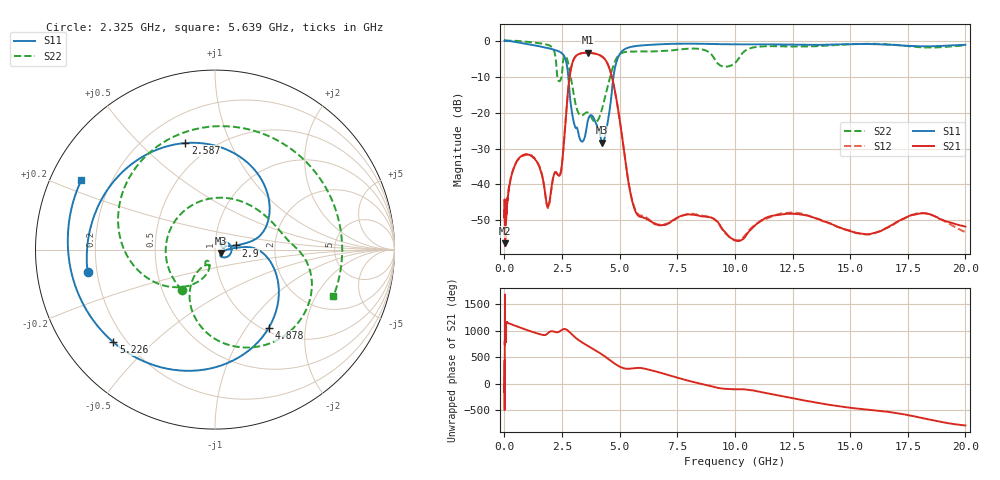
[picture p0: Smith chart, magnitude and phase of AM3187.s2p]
!Agilent Technologies,E8364B,MY43040894,A.07.50.67
!Agilent E8364B: A.07.50.67
!Date: Friday, December 27, 2019 08:39:41
!Correction: S11(Full 2 Port(1,2))
!S21(Full 2 Port(1,2))
!S12(Full 2 Port(1,2))
!S22(Full 2 Port(1,2))
!S2P File: Measurements: S11, S21, S12, S22:Log Frequency Sweep
# Hz S  dB  R 50
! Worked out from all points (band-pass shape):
!   3201 points, 10 MHz to 20 GHz, reference 50 ohm
!   highest |S21| = -3.33 dB at 3.608 GHz (marker M1); lowest = -56.4 dB at 25.98 MHz (marker M2)
!   |S21| within 3 dB of the highest: 2.942 GHz to 4.473 GHz (1.53 GHz wide, 41.3 % of centre)
!   lowest |S11| = -28.4 dB at 4.251 GHz (marker M3), VSWR 1.08, Z = 53.2 - j2.29 ohm
!   |S11| at or under -10 dB: 2.774 GHz to 4.732 GHz (1.957 GHz wide, 52.2 % of centre)
!   |S22| runs from -22.6 to 0.1 dB; largest |S21 - S12| = 0.011
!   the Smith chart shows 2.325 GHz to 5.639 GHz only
!   S11 on the Smith chart (normalised r, x): 2.325 GHz: 0.16, -0.09; 2.587 GHz: 0.36, +0.69; 2.9 GHz: 1.26, +0.06; 4.878 GHz: 1.06, -1.28; 5.226 GHz: 0.15, -0.38; 5.639 GHz: 0.09, +0.24
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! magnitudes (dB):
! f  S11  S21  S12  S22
! 10 MHz  0.1  -47.1  -44.2  0.0
! 25.98 MHz  0.0  -56.4  -53.9  0.0
! 35.55 MHz  0.0  -54.4  -55.6  0.1
! 47.61 MHz  0.0  -47.6  -48.1  0.1
! 126.1 MHz  0.0  -44.3  -44.6  0.0
! 447.2 MHz  -0.3  -34.7  -34.8  0.0
! 1.022 GHz  -1.0  -31.7  -31.6  -0.3
! 1.59 GHz  -1.6  -36.5  -36.3  -0.7
! 1.886 GHz  -2.0  -46.3  -46.6  -1.1
! 2.325 GHz  -2.8  -37.4  -37.3  -10.7
! 2.587 GHz  -4.2  -27.9  -27.9  -4.5
! 2.9 GHz  -18.6  -7.5  -7.5  -10.9
! 3.328 GHz  -27.9  -3.5  -3.5  -20.8
! 3.608 GHz  -22.6  -3.3  -3.3  -19.9
! 4.251 GHz  -28.4  -4.5  -4.4  -18.7
! 4.878 GHz  -5.5  -16.9  -17.0  -4.7
! 5.226 GHz  -2.3  -32.3  -32.3  -3.1
! 5.639 GHz  -1.5  -46.7  -46.4  -3.0
! 8.834 GHz  -0.9  -49.0  -49.0  -3.0
! 10.07 GHz  -1.0  -55.7  -55.5  -5.8
! 12.35 GHz  -1.1  -48.2  -47.9  -1.6
! 20 GHz  -1.1  -51.7  -53.3  -1.3
